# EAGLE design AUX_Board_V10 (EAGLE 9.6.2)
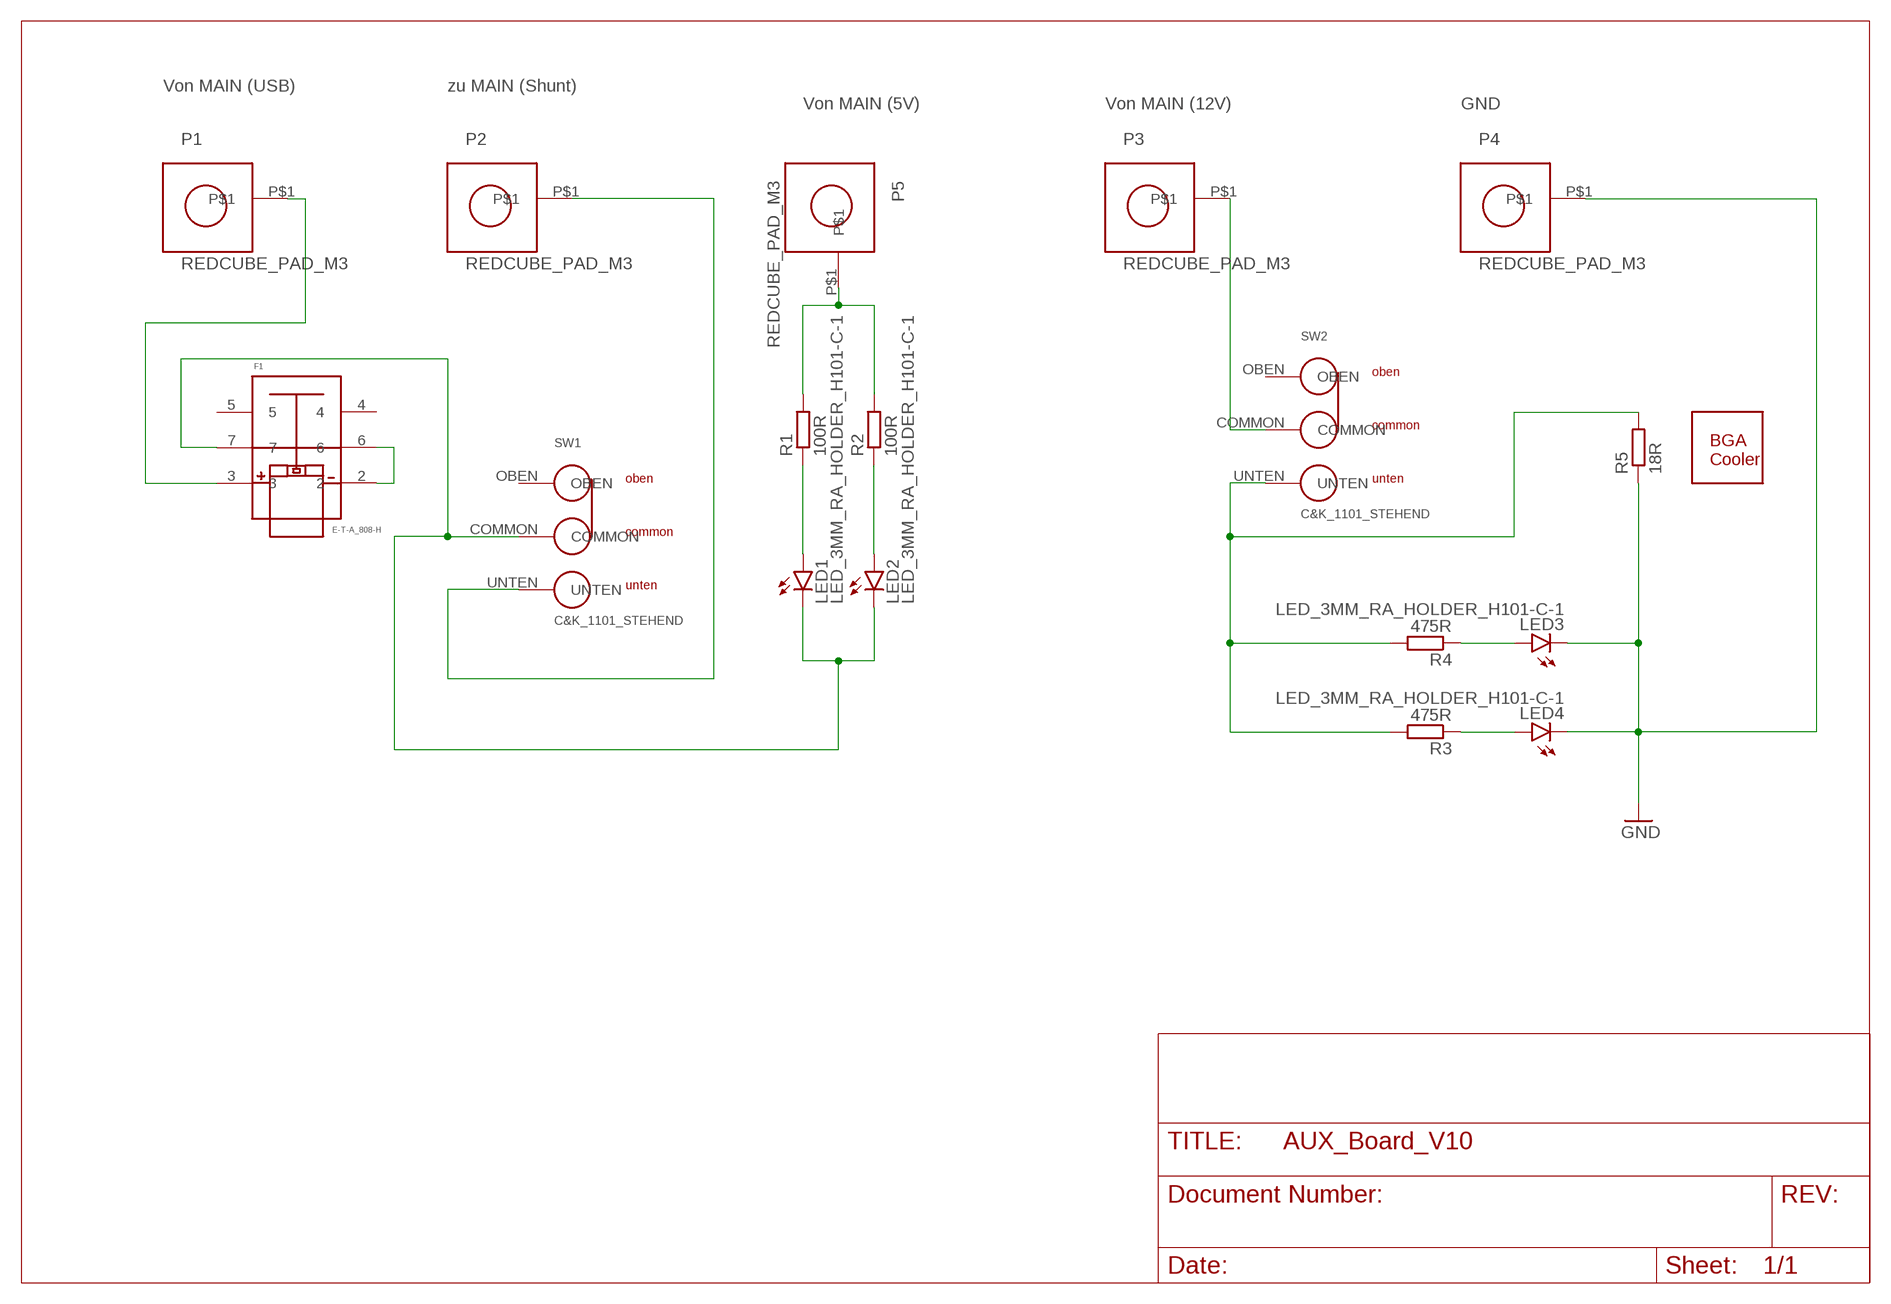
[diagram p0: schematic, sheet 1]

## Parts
F1  E-T-A_808-H  [E-T-A_808-H]
KK1  WAKEFIELD_VETTE_960_23X23_SIDE  [WAKEFIELD_VETTE_960_23X23_SIDE]
LED1  LED_3MM_RA_HOLDER_H101-C-1  [LED_3MM_RA_HOLDER_H101-C-1]
LED2  LED_3MM_RA_HOLDER_H101-C-1  [LED_3MM_RA_HOLDER_H101-C-1]
LED3  LED_3MM_RA_HOLDER_H101-C-1  [LED_3MM_RA_HOLDER_H101-C-1]
LED4  LED_3MM_RA_HOLDER_H101-C-1  [LED_3MM_RA_HOLDER_H101-C-1]
P1  REDCUBE_PAD_M3  [REDCUBE_PAD_M3]
P2  REDCUBE_PAD_M3  [REDCUBE_PAD_M3]
P3  REDCUBE_PAD_M3  [REDCUBE_PAD_M3]
P4  REDCUBE_PAD_M3  [REDCUBE_PAD_M3]
P5  REDCUBE_PAD_M3  [REDCUBE_PAD_M3]
R1  100R  R-EU_R1206  [R1206]
R2  100R  R-EU_R1206  [R1206]
R3  475R  R-EU_R1206  [R1206]
R4  475R  R-EU_R1206  [R1206]
R5  18R  R-EU_0204/5  [0204/5_DRILL_1MM]
SW1  C&K_1101_STEHEND  [C&K_1101_STEHEND]
SW2  C&K_1101_STEHEND  [C&K_1101_STEHEND]

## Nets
GND: LED3.P$2(C) LED4.P$2(C) P4.P$1 R5.1
N$1: F1.3 P1.P$1
N$2: F1.2 F1.6
N$3: F1.7 LED1.P$2(C) LED2.P$2(C) SW1.COMMON
N$4: P2.P$1 SW1.UNTEN
N$5: LED1.P$1(A) R1.1
N$6: LED2.P$1(A) R2.1
N$7: P5.P$1 R1.2 R2.2
N$8: P3.P$1 SW2.COMMON
N$9: R3.2 R4.2 R5.2 SW2.UNTEN
N$11: LED3.P$1(A) R4.1
N$12: LED4.P$1(A) R3.1
Unconnected: F1.4 F1.5 SW1.OBEN SW2.OBEN

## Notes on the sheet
- Von MAIN (USB) | zu MAIN (Shunt)
- Von MAIN (5V) | Von MAIN (12V) | GND

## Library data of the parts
F1 = Antec-Hood:E-T-A_808-H
KK1 = Antec-Hood:WAKEFIELD_VETTE_960_23X23_SIDE
LED1-LED4 = Antec-Hood:LED_3MM_RA_HOLDER_H101-C-1
P1-P5 = Antec-Hood:REDCUBE_PAD_M3
R1-R4 = rcl:R-EU_: RESISTOR, European symbol; SPICEPREFIX: R
R5 = Antec-Hood:R-EU_: RESISTOR, European symbol; SPICEPREFIX: R
SW1 SW2 = Antec-Hood:C&K_1101_STEHEND

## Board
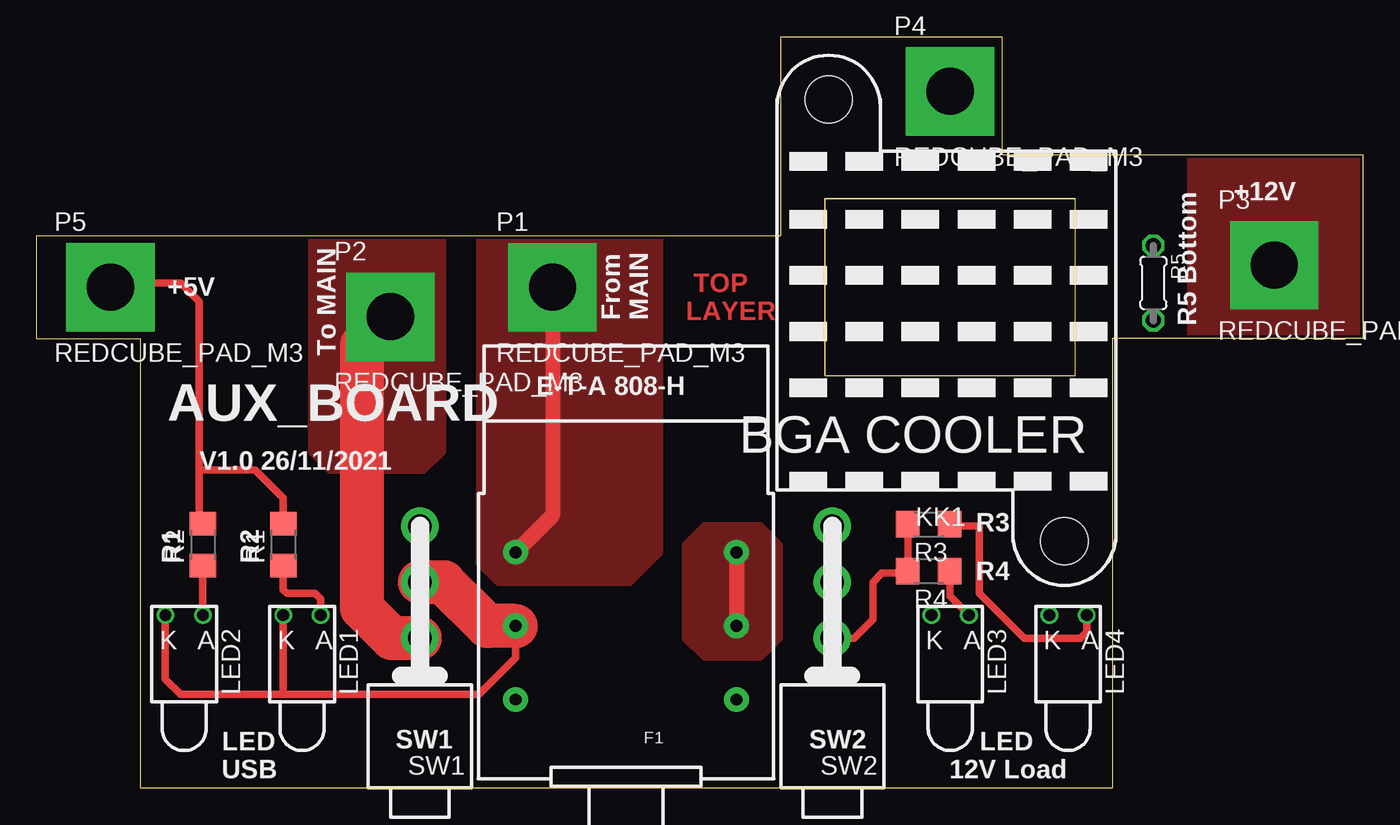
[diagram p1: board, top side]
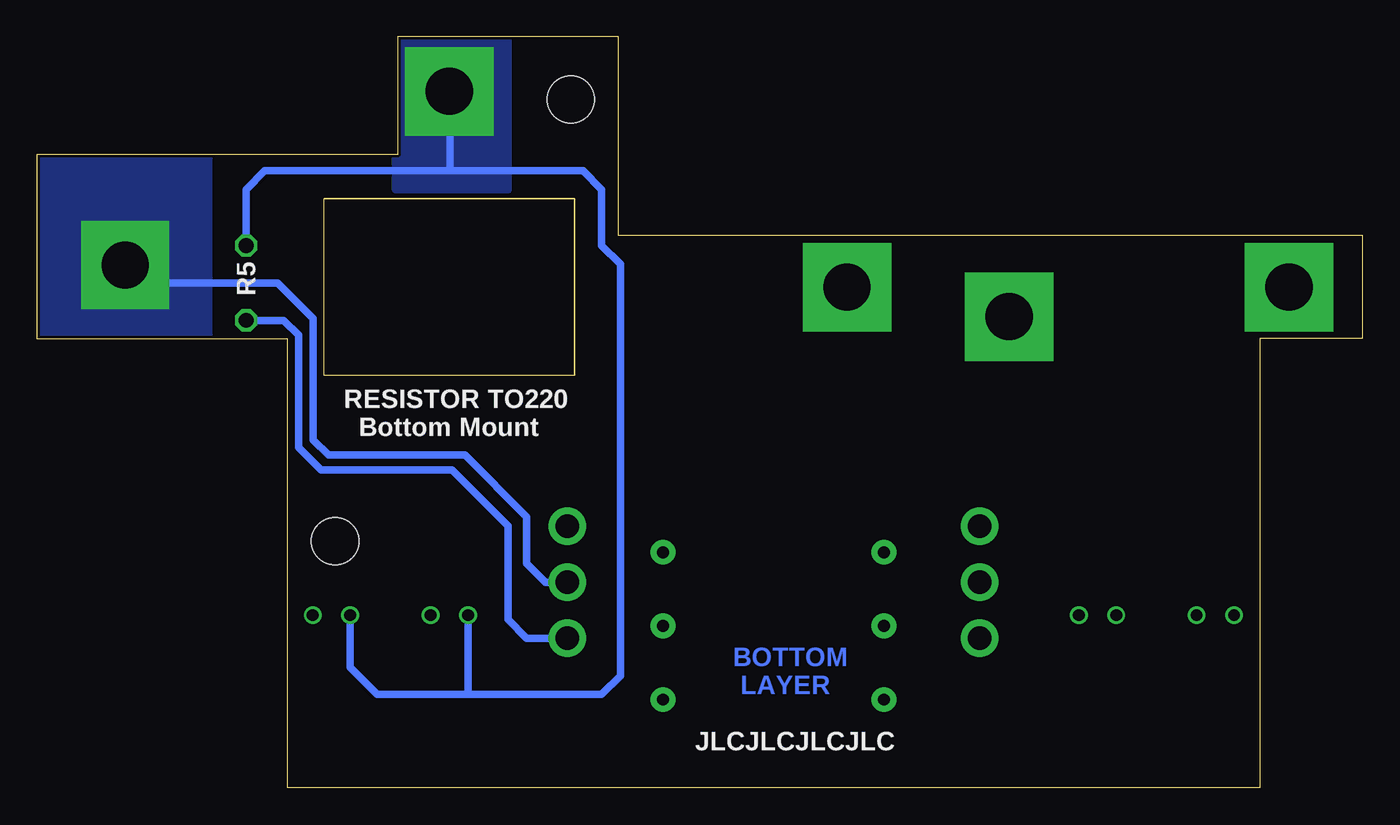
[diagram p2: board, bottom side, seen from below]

Size 90 x 51 mm. Coordinates in mm from the lower left corner, seen from the top.
Outline: 7,0 73,0 73,30.5 90,30.5 90,43 65.5,43 65.5,51 50.5,51 50.5,37.5 0,37.5 0,30.5 7,30.5 7,0
Outline: 53.5,28 70.5,28 70.5,40 53.5,40 53.5,28
Copper layers (1*16): Top 0.035mm / dielectric 1.5mm / Bottom 0.035mm
Design rules "JLCPCB_2alyer": minimum track width 5mil, minimum drill 0.2mm, track to track 5mil, track to pad 0.2mm, pad to pad 0.2mm, via to via 0.2mm, smd to smd 5mil, copper to edge 0.2mm, drill to drill 0.5mm, minimum pad ring 0.13mm, minimum via ring 0.13mm, stop-mask expansion 0.05mm, vias tented up to drill 0mil, thermal gap 10mil
Milling: 4 lines

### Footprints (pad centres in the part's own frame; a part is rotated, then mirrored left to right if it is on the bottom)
E-T-A_808-H = drill 0.8 pad 1.676: 2 -7.5,-16; 3 7.5,-16; 4 -7.5,-6; 5 7.5,-6; 6 -7.5,-11; 7 7.5,-11
WAKEFIELD_VETTE_960_23X23_SIDE = hole 3.2: -15,-8; 15,8
LED_3MM_RA_HOLDER_H101-C-1 = drill 0.8: P$1 -1.27,-9.2; P$2 1.27,-9.2
REDCUBE_PAD_M3 = drill 3.2 pad 6 square: P$1 0,0
R1206 = smd 1.6 x 1.803: 1 -1.422,0; 2 1.422,0
0204/5_DRILL_1MM = drill 1 octagon: 1 -2.54,0; 2 2.54,0
C&K_1101_STEHEND = drill 1.6 pad 2.54: COMMON 0,-13.97; OBEN 0,-17.78; UNTEN 0,-10.16

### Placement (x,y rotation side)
F1  40,0 180 top
KK1  61.75,31.75 90 top
LED1  18,2.54 180 top
LED2  10,2.54 180 top
LED3  62,2.54 180 top
LED4  70,2.54 180 top
P1  35,34 0 top
P2  24,32 0 top
P3  84,35.5 0 top
P4  62,47.3 0 top
P5  5,34 0 top
R1  16.73,16.51 90 top
R2  11.27,16.51 90 top
R3  60.55,17.91 180 top
R4  60.55,14.73 180 top
R5  75.79,34.29 270 top
SW1  26,0 180 top
SW2  54,0 180 top

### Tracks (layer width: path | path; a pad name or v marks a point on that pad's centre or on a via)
GND
  Bottom 0.5: R5.1 75.79,40.64 74.52,41.91 61.95,41.91 | 61.95,41.91 61.95,47.25 P4.P$1 | LED4.P$2 68.73,8.18 66.9,6.35 60.55,6.35 | 60.55,6.35 51.66,6.35 50.39,7.62 50.39,35.56 51.66,36.83 51.66,40.64 52.93,41.91 61.95,41.91 | LED3.P$2 60.73,6.53 60.55,6.35
  pour Bottom (no thermals): 58.01,50.8 58.01,40.64 65.63,40.64 65.63,50.8
N$1
  Top 1.016: P1.P$1 35,18.5 F1.3
  pour Top (no thermals): 30.07,39.37 30.07,15.24 31.34,13.97 40.23,13.97 42.26,16 42.26,39.37
N$2
  Top 1.016: F1.2 F1.6
  pour Top: 44.04,16.51 44.04,10.16 45.31,8.89 49.12,8.89 50.39,10.16 50.39,16.51 49.12,17.78 45.31,17.78
N$3
  Top 0.508: F1.7 32.5,8.84 30.01,6.35 16.73,6.35 | LED2.P$2 8.73,7.37 9.75,6.35 16.73,6.35 | LED1.P$2 16.73,6.36 16.73,6.35
  Top 3: F1.7 30.59,11 27.62,13.97 SW1.COMMON
N$4
  Top 3: SW1.UNTEN 24.1,10.16 22.07,12.19 22.07,30.07 P2.P$1
  pour Top (no thermals): 17.37,39.37 18.64,38.1 18.64,22.86 19.91,21.59 26.26,21.59 27.53,22.86 27.53,39.37
N$5
  Top 0.508: R1.1 16.73,13.46 16.99,13.21 18.89,13.21 19.27,12.83 LED1.P$1
N$6
  Top 0.508: LED2.P$1 R2.1
N$7
  Top 0.508: R1.2 16.73,19.68 14.83,21.59 11.02,21.59 | P5.P$1 5.29,34.29 9.75,34.29 11.02,33.02 11.02,21.59 | R2.2 11.02,18.19 11.02,21.59
N$8
  Bottom 0.5: SW2.COMMON 55.47,13.97 56.74,15.24 56.74,18.41 60.93,22.61 70.2,22.61 71.23,23.63 71.23,31.88 73.64,34.29 82.79,34.29 P3.P$1
  pour Bottom (no thermals): 78.33,44.45 78.33,29.21 79.6,27.94 91.03,27.94 92.3,29.21 92.3,44.45
  pour Top (no thermals): 78.33,45.72 78.33,27.94 79.6,26.67 92.3,26.67 93.57,27.94 93.57,45.72
N$9
  Top 0.5: 57.38,14.61 56.74,13.97 56.74,11.43 55.47,10.16 SW2.UNTEN
  Top 0.508: 57.38,14.61 59,14.61 R4.2 R3.2
  Bottom 0.5: SW2.UNTEN 56.74,10.16 58.01,11.43 58.01,17.78 61.82,21.59 70.71,21.59 72.23,23.11 72.23,30.73 73.25,31.75 R5.2
N$11
  Top 0.508: R4.1 61.97,13.04 LED3.P$1
N$12
  Top 0.508: R3.1 62.1,17.78 63.98,17.78 63.98,13.21 67.03,10.16 70.84,10.16 71.27,10.59 LED4.P$1

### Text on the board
Top: TOP / LAYER
Bottom: BOTTOM / LAYER
tPlace: +12V | +5V | From / MAIN | R5 Bottom | To MAIN | E-T-A 808-H | AUX_BOARD | V1.0 26/11/2021 | R3 | R1 | R2 | R4 | SW1 | SW2 | LED / USB | LED / 12V Load
bPlace: R5 | RESISTOR TO220 / Bottom Mount | JLCJLCJLCJLC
